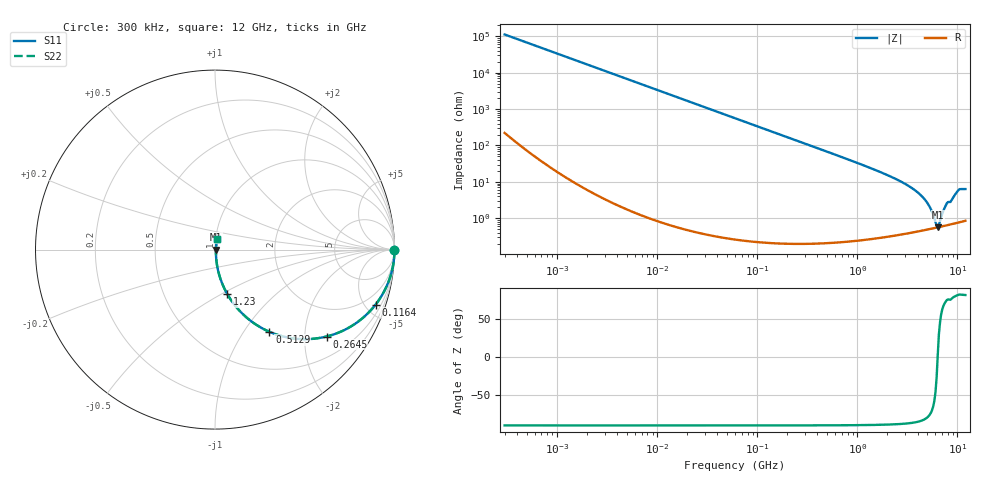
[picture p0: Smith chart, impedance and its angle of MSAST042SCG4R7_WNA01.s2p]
! MSAST042SCG4R7_WNA01  S-PARAMETER MODEL  ( General Type )
! Model Generated by TAIYO YUDEN Corporation (http://www.ty-top.com)
! Version 1.0
! TAIYO YUDEN Control No. 150820
! Copyright(c) 2015 TAIYO YUDEN CO.,LTD. All Rights Reserved.
! Product Description (link to TY-COMPAS)
! https://ds.yuden.co.jp/TYCOMPAS/or/detail?pn=MSAST042SCG4R7BWNA01&u=M
! Products Name : Multilayer Ceramic Capacitors
! Characteristics :
!  Capacitance : 4.7 pF , Rated Voltage : 25V , TCC : CG / C0G
!  Case Size : 0.4 x 0.2 / 0.016 x 0.008 [mm/inch] , Thickness : 0.2 / 0.008 [mm/inch]
!  (Conditions: Temperature = 25 degC , DC Bias Current/Voltage = 0A / 0V)
! External Node Assignments :
!  1  o---| |---o  2
! GND o---------o GND
! Frequency Range : 0.3MHz  -  12000MHz  [ 401 STEP ]
# MHz S RI R 50
! Freq[MHz].  S11 Real  S11 Imag  S21 Real  S21 Imag  S12 Real  S12 Imag  S22 Real  S22 Imag
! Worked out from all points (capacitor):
!   401 points, 300 kHz to 12 GHz, reference 50 ohm
!   read as one part in series: C = 4.69 pF near 316.3 kHz
!   lowest |Z| = 561 mohm at 6.354 GHz (marker M1)
!   series resonance near 6.339 GHz, so ESL is about 130 pH
!   S11 on the Smith chart (normalised r, x): 300 kHz: open; 116.4 MHz: 1.00, -5.84; 264.5 MHz: 1.00, -2.56; 512.9 MHz: 1.00, -1.32; 1.23 GHz: 1.01, -0.53; 12 GHz: 1.02, +0.13
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0.3  1 -0.000883  2.51e-06 0.000883  2.51e-06 0.000883  1 -0.000883
1.769972  1 -0.00521  2.91e-05 0.00521  2.91e-05 0.00521  1 -0.00521
10.44266  0.999 -0.0307  0.000952 0.0307  0.000952 0.0307  0.999 -0.0307
60  0.9697 -0.1713  0.0303 0.1713  0.0303 0.1713  0.9697 -0.1713
116.3536  0.8948 -0.3065  0.1052 0.3065  0.1052 0.3065  0.8948 -0.3065
264.5085  0.6215 -0.4842  0.3785 0.4842  0.3785 0.4842  0.6215 -0.4842
353.9943  0.4779 -0.4985  0.5221 0.4985  0.5221 0.4985  0.4779 -0.4985
512.9422  0.3027 -0.4578  0.6973 0.4578  0.6973 0.4578  0.3027 -0.4578
783.7017  0.1554 -0.3597  0.8446 0.3597  0.8446 0.3597  0.1554 -0.3597
1229.528  0.0681 -0.2472  0.9319 0.2472  0.9319 0.2472  0.0681 -0.2472
2088.533  0.0235 -0.1412  0.9765 0.1412  0.9765 0.1412  0.0235 -0.1412
3276.641  0.00955 -0.0751  0.9904 0.0751  0.9904 0.0751  0.00955 -0.0751
4385.161  0.00612 -0.0402  0.9939 0.0402  0.9939 0.0402  0.00612 -0.0402
5140.631  0.00543 -0.0226  0.9946 0.0226  0.9946 0.0226  0.00543 -0.0226
5565.855  0.00535 -0.0141  0.9947 0.0141  0.9947 0.0141  0.00535 -0.0141
6026.253  0.00543 -0.00565  0.9946 0.00565  0.9946 0.00565  0.00543 -0.00565
6354.153  0.00557 0.000291  0.9944 -0.000291  0.9944 -0.000291  0.00557 0.000291
6699.894  0.00579 0.00605  0.9942 -0.00605  0.9942 -0.00605  0.00579 0.00605
7254.098  0.00627 0.0151  0.9937 -0.0151  0.9937 -0.0151  0.00627 0.0151
7854.144  0.00698 0.0249  0.993 -0.0249  0.993 -0.0249  0.00698 0.0249
10236.47  0.0109 0.0575  0.9891 -0.0575  0.9891 -0.0575  0.0109 0.0575
12000  0.0122 0.0615  0.9878 -0.0615  0.9878 -0.0615  0.0122 0.0615
